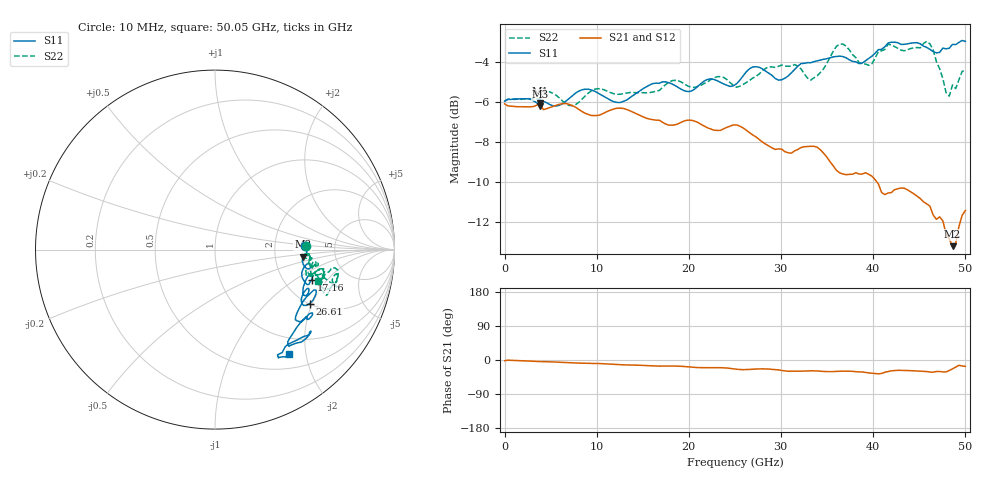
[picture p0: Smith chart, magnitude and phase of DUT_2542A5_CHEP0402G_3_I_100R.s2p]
! 11/3/2025 4:14:19 PM
! C:\MESURES\046-TRL-DUT-CHEP\0402\DUT-2542A5-CHEP0402G-3-I.S2P
! CHANNEL.1 Sparams
! TR.MEASUREMENT
! CORRECTED.DATA
! RF.CORRECTION: CAL.A: FULL.TWO.PORT.CALCAL.A: Port 1,4
! AVERAGING.OFF
! IF.BANDWIDTH: 500HZ
! SWEEPTYPE:  FREQ.SWEEP(Linear)
! Reference Plane Port Info
! PORT:  PORT1  PORT4
! DISTANCE:  0  m  0  m
! TIME:  0  s  0  s
! PHASE.OFFSET:  0  deg.  0  deg.
! LOSS:  0  dB  0  dB
! REF.LOSS:  0  dB  0  dB
! REF.FREQ:  0  Hz  0  Hz
! Power Info
! POWER:  -10  dBm  -10  dBm
! EFF.POWER:  -10  dBm  -10  dBm
! SOURCE.ATTEN:  0  dB  0  dB
! TEST.ATTEN:  0  dB  0  dB
! PORTZ: Port1:50 Port4:50
# GHZ S RI R 50
! FREQ.GHZ  S11RE  S11IM  S41RE  S41IM  S14RE  S14IM  S44RE  S44IM
!; PortSelection: Port_14 (1-->1,4-->4)
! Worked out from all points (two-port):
!   144 points, 10 MHz to 50.05 GHz, reference 50 ohm
!   highest |S21| = -6.04 dB at 3.859 GHz (marker M1); lowest = -13.2 dB at 48.65 GHz (marker M2)
!   |S21| within 3 dB of the highest: start of sweep to 35.47 GHz
!   lowest |S11| = -6.2 dB at 3.859 GHz (marker M3), VSWR 2.92, Z = 144 - j14.8 ohm
!   |S11| at or under -10 dB: nowhere
!   |S22| runs from -6.2 to -3.0 dB; largest |S21 - S12| = 0.0052
!   S11 on the Smith chart (normalised r, x): 10 MHz: 3.03, +0.14; 17.16 GHz: 2.83, -1.39; 26.61 GHz: 2.01, -1.92; 50.05 GHz: 0.72, -1.70
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0.01  0.5041 0.0173  0.4963 -0.0164  0.4967 -0.0171  0.5044 0.0173
3.85945  0.4887 -0.0389  0.4973 -0.0364  0.4959 -0.0353  0.5087 -0.0335
8.4088  0.528 -0.1056  0.4702 -0.0692  0.4693 -0.0675  0.5073 -0.0491
16.8076  0.5297 -0.1797  0.4341 -0.1257  0.4339 -0.1226  0.5294 -0.0881
17.15755  0.5384 -0.1677  0.4293 -0.1232  0.429 -0.1206  0.5371 -0.0962
18.9073  0.5278 -0.1356  0.4255 -0.1242  0.4263 -0.1224  0.5625 -0.0707
21.007  0.4912 -0.2474  0.4191 -0.1531  0.4197 -0.1507  0.5412 -0.0938
23.8066  0.5125 -0.218  0.4027 -0.1515  0.4037 -0.1487  0.5732 -0.0755
25.2064  0.4802 -0.2836  0.4007 -0.1814  0.4014 -0.1789  0.5338 -0.1169
26.6062  0.5281 -0.301  0.3816 -0.177  0.3832 -0.1741  0.5531 -0.1307
28.35595  0.5564 -0.224  0.3611 -0.157  0.362 -0.1544  0.5988 -0.1118
31.15555  0.4474 -0.3906  0.3253 -0.1839  0.3271 -0.181  0.5994 -0.1441
33.6052  0.5121 -0.3725  0.3414 -0.1861  0.3435 -0.184  0.5597 -0.1403
35.7049  0.524 -0.3867  0.2988 -0.177  0.2993 -0.1747  0.6361 -0.2195
37.8046  0.5218 -0.361  0.2873 -0.1645  0.2875 -0.1626  0.6514 -0.1005
40.6042  0.4121 -0.5392  0.2517 -0.1861  0.2526 -0.1832  0.6206 -0.2554
42.004  0.5004 -0.5016  0.2614 -0.1426  0.2625 -0.1401  0.6811 -0.1485
44.8036  0.5247 -0.4733  0.2548 -0.1417  0.2554 -0.1384  0.6587 -0.1955
46.2034  0.4552 -0.5051  0.2337 -0.1455  0.2347 -0.1409  0.6722 -0.2014
47.95315  0.3486 -0.5862  0.2003 -0.1223  0.2014 -0.1187  0.5087 -0.1476
48.65305  0.3535 -0.604  0.2008 -0.0866  0.2012 -0.0838  0.5338 -0.1479
50.05285  0.4129 -0.5799  0.2572 -0.0777  0.2585 -0.0733  0.5752 -0.1757
